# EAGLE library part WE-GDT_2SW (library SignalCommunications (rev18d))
SMD Gate Drive Transformer WE-GDT Characteristics - small form factor EP5 - 1 or 2 secondary windings - 4 different turn rations - 1500VDC insulation test voltage - operating voltage up to 80V Applications -- Gate Drive -- Signal -- Power -- Synchronous Flyback Details see: http://katalog.we-online.de/en/pbs/WE-GDT? Updated by Dan Xu 2014-05-19 2014 (C) Wurth Elektronik
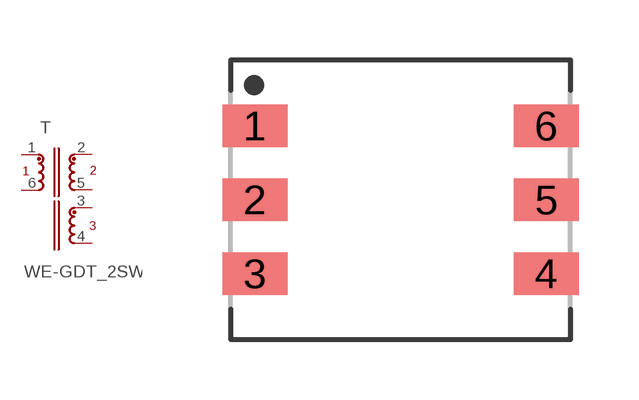
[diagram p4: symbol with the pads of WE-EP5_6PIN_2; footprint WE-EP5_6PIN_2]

Designator prefix T

## WE-GDT_2SW_760301105  [WE-EP5_6PIN_2]
1  1  pas
2  2  pas
3  4  pas
4  5  pas
5  3  pas
6  6  pas

## WE-GDT_2SW_760301104  [WE-EP5_6PIN_2]
Pads as for WE-EP5_6PIN_2

## WE-GDT_2SW_760301103  [WE-EP5_6PIN_2]
Pads as for WE-EP5_6PIN_2

## Footprint WE-EP5_6PIN_2 (pad centres in mm)
smd 1.63 x 1.07: 1 -3.645,1.85; 2 -3.645,0; 3 -3.645,-1.85; 4 3.645,-1.85; 5 3.645,0; 6 3.645,1.85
